[IBIS Ver]   4.2
[File Name]  stm32f2_lqfp100.ibs
[File Rev]   1.0
[Date]   31-Aug-2011
[Source]   STMicroelectronics NV
[Notes]   The I/O models have been made by simulation and qualified
   with recomandation of QualityIBIS flow.
   Some Models, library and pin names may be modified.
   Details of modified names can be found below.
ORIGINAL NAME   ::  MODIFIED NAME   :: COMMENTS(if any)
IO8USB_LSFS_OTG_FT  ::  IO8USB_LSFS_OTG_FT_USB   :: Model in USB mode.
IO8USB_LSFS_OTG_FT  ::  IO8USB_LSFS_OTG_FT_NON_USB_DNV33  :: Model in other than USB mode & pad pin = DNV33
IO8USB_LSFS_OTG_FT  ::  IO8USB_LSFS_OTG_FT_NON_USB_DPV33  :: Model in other than USB mode & pad pin = DPV33
[Disclaimer] These IBIS models are the proprietary information of
   STMicroelectronics and are disclosed to users solely for
   modeling and simulation purposes. No further license is
   implied. All warranties express, implied, or statutory,
   including any implied warranty of fitness for a particular
   purpose or implied warranty against infringement, are
   hereby disclaimed. STMicroelectronics reserves the right
   to change the IBIS models at any time and without notice.
[Copyright]  (c) STMicroelectronics
   All rights reserved. Reproduction in whole or part is prohibited
   without the written consent of the copyright holder.
[Component]  STM32F2_LQFP100
[Manufacturer] STMicroelectronics NV
[Package]
| variable   typ   min   max
R_pkg   0.000mOhm   0.000mOhm   0.000mOhm
L_pkg   0.000nH   0.000nH   0.000nH
C_pkg   0.000pF   0.000pF   0.000pF
[Pin]   signal_name   model_name
1 PE2 IO8PROG2M25M50M100M_ARSUDQ_FT
2 PE3 IO8PROG2M25M50M100M_ARSUDQ_FT
3 PE4 IO8PROG2M25M50M100M_ARSUDQ_FT
4 PE5 IO8PROG2M25M50M100M_ARSUDQ_FT
5 PE6 IO8PROG2M25M50M100M_ARSUDQ_FT
|6 VBAT VDD33IOSWCO_MOSSWI_FT
7 PC13 IO8PROG2M25M50M100M_ARWSUDQ_FT_V33
8 PC14 IO8PROG2M25M50M100M_ARWSUDQ_FT
9 PC15 IO8PROG2M25M50M100M_ARSUDQ_FT
|10 VSS_5 VSSIOCO
|11 VDD_5 VDD33IOCO
12 PH0 IO8PROG2M25M50M100M_ARSUDQ_FT
13 PH1 IO8PROG2M25M50M100M_ARSUDQ_FT
|14 NRST RESET
15 PC0 IO8PROG2M25M50M100M_AR3WSUDQ_FT
16 PC1 IO8PROG2M25M50M100M_AR3WSUDQ_FT
17 PC2 IO8PROG2M25M50M100M_AR3WSUDQ_FT
18 PC3 IO8PROG2M25M50M100M_AR3WSUDQ_FT
|19 VDD_12 VDD33IOCO_VSSIOCO_MOSSWI_FT
|20 VSSA VSSCO
|21 VREF+ VDD33CO
|22 VDDA VDD33CO
23 PA0 IO8PROG2M25M50M100M_AR3WSUDQ_FT_V33
24 PA1 IO8PROG2M25M50M100M_AR3WSUDQ_FT
25 PA2 IO8PROG2M25M50M100M_AR3WSUDQ_FT
26 PA3 IO8PROG2M25M50M100M_AR3WSUDQ_FT
|27 VSS_4 VSSIOCO
|28 VDD_4 VDD33IOCO
29 PA4 IO8PROG2M25M50M100M_AR3WSUDQ_FT
30 PA5 IO8PROG2M25M50M100M_AR3WSUDQ_FT
31 PA6 IO8PROG2M25M50M100M_AR3WSUDQ_FT
32 PA7 IO8PROG2M25M50M100M_AR3WSUDQ_FT
33 PC4 IO8PROG2M25M50M100M_AR3WSUDQ_FT
34 PC5 IO8PROG2M25M50M100M_AR3WSUDQ_FT
35 PB0 IO8PROG2M25M50M100M_AR3WSUDQ_FT
36 PB1 IO8PROG2M25M50M100M_AR3WSUDQ_FT
37 PB2 IO8PROG2M25M50M100M_AR3WSUDQ_FT
38 PE7 IO8PROG2M25M50M100M_ARSUDQ_FT
39 PE8 IO8PROG2M25M50M100M_ARSUDQ_FT
40 PE9 IO8PROG2M25M50M100M_ARSUDQ_FT
41 PE10 IO8PROG2M25M50M100M_ARSUDQ_FT
42 PE11 IO8PROG2M25M50M100M_ARSUDQ_FT
43 PE12 IO8PROG2M25M50M100M_ARSUDQ_FT
44 PE13 IO8PROG2M25M50M100M_ARSUDQ_FT
45 PE14 IO8PROG2M25M50M100M_ARSUDQ_FT
46 PE15 IO8PROG2M25M50M100M_ARSUDQ_FT
47 PB10 IO8PROG2M25M50M100M_ARSUDQ_I2CIN_FT
48 PB11 IO8PROG2M25M50M100M_ARSUDQ_I2CIN_FT
|49 VCAP1_0
|50 VDD_1
51 PB12 IO8USB_ID_OTG_FT
52 PB13 IO8USB_VBUS_OTG_FT
|53 PA11 IO8USB_LSFS_OTG_FT_USB
53 PA11 IO8USB_LSFS_OTG_FT_NON_USB_DNV33
|54 PA12 IO8USB_LSFS_OTG_FT_USB
54 PA12 IO8USB_LSFS_OTG_FT_NON_USB_DPV33
55 PD8 IO8PROG2M25M50M100M_ARSUDQ_FT
56 PD9 IO8PROG2M25M50M100M_ARSUDQ_FT
57 PD10 IO8PROG2M25M50M100M_ARSUDQ_FT
58 PD11 IO8PROG2M25M50M100M_ARSUDQ_FT
59 PD12 IO8PROG2M25M50M100M_ARSUDQ_FT
60 PD13 IO8PROG2M25M50M100M_ARSUDQ_FT
61 PD14 IO8PROG2M25M50M100M_ARSUDQ_FT
62 PD15 IO8PROG2M25M50M100M_ARSUDQ_FT
63 PC6 IO8PROG2M25M50M100M_ARSUDQ_FT
64 PC7 IO8PROG2M25M50M100M_ARSUDQ_FT
65 PC8 IO8PROG2M25M50M100M_ARSUDQ_FT
66 PC9 IO8PROG2M25M50M100M_ARSUDQ_I2CIN_FT
67 PA8 IO8PROG2M25M50M100M_ARSUDQ_I2CIN_FT
68 PA9 IO8USB_VBUS_OTG_FT
69 PA10 IO8USB_ID_OTG_FT
70 PA11 IO8USB_LSFS_OTG_FT_USB
|70 PA11 IO8USB_LSFS_OTG_FT_NON_USB_DNV33
71 PA12 IO8USB_LSFS_OTG_FT_USB
|71 PA12 IO8USB_LSFS_OTG_FT_NON_USB_DPV33
72 PA13 IO8PROG2M25M50M100M_ARSUDQ_FT
|73 VCAP2
|74 VSS_2
|75 VDD_2
76 PA14 IO8PROG2M25M50M100M_ARSUDQ_FT
77 PA15 IO8PROG2M25M50M100M_AR3WSUDQ_FT
78 PC10 IO8PROG2M25M50M100M_ARSUDQ_FT
79 PC11 IO8PROG2M25M50M100M_ARSUDQ_FT
80 PC12 IO8PROG2M25M50M100M_ARSUDQ_FT
81 PD0 IO8PROG2M25M50M100M_ARSUDQ_FT
82 PD1 IO8PROG2M25M50M100M_ARSUDQ_FT
83 PD2 IO8PROG2M25M50M100M_ARSUDQ_FT
84 PD3 IO8PROG2M25M50M100M_ARSUDQ_FT
85 PD4 IO8PROG2M25M50M100M_ARSUDQ_FT
86 PD5 IO8PROG2M25M50M100M_ARSUDQ_FT
87 PD6 IO8PROG2M25M50M100M_ARSUDQ_FT
88 PD7 IO8PROG2M25M50M100M_ARSUDQ_FT
89 PB3 IO8PROG2M25M50M100M_ARSUDQ_FT
90 PB4 IO8PROG2M25M50M100M_ARSUDQ_FT
91 PB5 IO8PROG2M25M50M100M_AR3WSUDQ_FT
92 PB6 IO8PROG2M25M50M100M_ARSUDQ_I2CIN_FT
93 PB7 IO8PROG2M25M50M100M_ARSUDQ_I2CIN_FT
94 BOOT0 VPP_TEST_HV
95 PB8 IO8PROG2M25M50M100M_ARSUDQ_I2CIN_FT
96 PB9 IO8PROG2M25M50M100M_ARSUDQ_I2CIN_FT
97 PE0 IO8PROG2M25M50M100M_ARSUDQ_FT
98 PE1 IO8PROG2M25M50M100M_ARSUDQ_FT
|99 NC
|100 VDD_3  VDD33CO
[Diff Pin]  inv_pin   vdiff tdelay_typ tdelay_min tdelay_max
|53 54 200mV 0  0 0
70 71 200mV 0  0 0
[Model Selector] IO8PROG2M25M50M100M_AR3WSUDQ_FT_V33
IO8PROG2M25M50M100M_AR3WSUDQ_DRV_V33_00   DRIVER MODEL  : SPEEDAV33=0 SPEEDBV33=0
IO8PROG2M25M50M100M_AR3WSUDQ_DRV_V33_01   DRIVER MODEL  : SPEEDAV33=0 SPEEDBV33=1
IO8PROG2M25M50M100M_AR3WSUDQ_DRV_V33_10   DRIVER MODEL  : SPEEDAV33=1 SPEEDBV33=0
IO8PROG2M25M50M100M_AR3WSUDQ_DRV_V33_11   DRIVER MODEL  : SPEEDAV33=1 SPEEDBV33=1
IO8PROG2M25M50M100M_AR3WSUDQ_RCV_V33_0   CMOS RECIEVER : ENHYSV33=0  OUTPUT=ZIV33
IO8PROG2M25M50M100M_AR3WSUDQ_RCV_V33_0_T  TTL  RECIEVER : ENHYSV33=0  OUTPUT=ZIV33
IO8PROG2M25M50M100M_AR3WSUDQ_RCV_V33_1   CMOS RECIEVER : ENHYSV33=1  OUTPUT=ZIV33
IO8PROG2M25M50M100M_AR3WSUDQ_RCV_V33_1_T  TTL  RECIEVER : ENHYSV33=1  OUTPUT=ZIV33
[Model Selector] IO8PROG2M25M50M100M_AR3WSUDQ_FT
IO8PROG2M25M50M100M_AR3WSUDQ_FT_DRV_00   DRIVER MODEL  : SPEEDAV12=0 SPEEDBV12=0
IO8PROG2M25M50M100M_AR3WSUDQ_FT_DRV_01   DRIVER MODEL  : SPEEDAV12=0 SPEEDBV12=1
IO8PROG2M25M50M100M_AR3WSUDQ_FT_DRV_10   DRIVER MODEL  : SPEEDAV12=1 SPEEDBV12=0
IO8PROG2M25M50M100M_AR3WSUDQ_FT_DRV_11   DRIVER MODEL  : SPEEDAV12=1 SPEEDBV12=1
IO8PROG2M25M50M100M_AR3WSUDQ_FT_RCV_00   CMOS RECIEVER : ENHYSV12=0  OUTPUT=ZIV12
IO8PROG2M25M50M100M_AR3WSUDQ_FT_RCV_00_T  TTL  RECIEVER : ENHYSV12=0  OUTPUT=ZIV12
IO8PROG2M25M50M100M_AR3WSUDQ_FT_RCV_01   CMOS RECIEVER : ENHYSV12=0  OUTPUT=ZIV33
IO8PROG2M25M50M100M_AR3WSUDQ_FT_RCV_01_T  TTL  RECIEVER : ENHYSV12=0  OUTPUT=ZIV33
IO8PROG2M25M50M100M_AR3WSUDQ_FT_RCV_10   CMOS RECIEVER : ENHYSV12=1  OUTPUT=ZIV12
IO8PROG2M25M50M100M_AR3WSUDQ_FT_RCV_10_T  TTL  RECIEVER : ENHYSV12=1  OUTPUT=ZIV12
IO8PROG2M25M50M100M_AR3WSUDQ_FT_RCV_11   CMOS RECIEVER : ENHYSV12=1  OUTPUT=ZIV33
IO8PROG2M25M50M100M_AR3WSUDQ_FT_RCV_11_T  TTL  RECIEVER : ENHYSV12=1  OUTPUT=ZIV33
[Model Selector] IO8PROG2M25M50M100M_ARSUDQ_FT
IO8PROG2M25M50M100M_ARSUDQ_FT_DRV_00   DRIVER MODEL  : SPEEDAV12=0 SPEEDBV12=0
IO8PROG2M25M50M100M_ARSUDQ_FT_DRV_01   DRIVER MODEL  : SPEEDAV12=0 SPEEDBV12=1
IO8PROG2M25M50M100M_ARSUDQ_FT_DRV_10   DRIVER MODEL  : SPEEDAV12=1 SPEEDBV12=0
IO8PROG2M25M50M100M_ARSUDQ_FT_DRV_11   DRIVER MODEL  : SPEEDAV12=1 SPEEDBV12=1
IO8PROG2M25M50M100M_ARSUDQ_FT_RCV_00   CMOS RECIEVER : ENHYSV12=0  OUTPUT=ZIV12
IO8PROG2M25M50M100M_ARSUDQ_FT_RCV_00_T   TTL  RECIEVER : ENHYSV12=0  OUTPUT=ZIV12
IO8PROG2M25M50M100M_ARSUDQ_FT_RCV_01   CMOS RECIEVER : ENHYSV12=0  OUTPUT=ZIV33
IO8PROG2M25M50M100M_ARSUDQ_FT_RCV_01_T   TTL  RECIEVER : ENHYSV12=0  OUTPUT=ZIV33
IO8PROG2M25M50M100M_ARSUDQ_FT_RCV_10   CMOS RECIEVER : ENHYSV12=1  OUTPUT=ZIV12
IO8PROG2M25M50M100M_ARSUDQ_FT_RCV_10_T   TTL  RECIEVER : ENHYSV12=1  OUTPUT=ZIV12
IO8PROG2M25M50M100M_ARSUDQ_FT_RCV_11   CMOS RECIEVER : ENHYSV12=1  OUTPUT=ZIV33
IO8PROG2M25M50M100M_ARSUDQ_FT_RCV_11_T   TTL  RECIEVER : ENHYSV12=1  OUTPUT=ZIV33
[Model Selector] IO8PROG2M25M50M100M_ARSUDQ_I2CIN_FT
IO8PROG2M25M50M100M_ARSUDQ_I2CIN_DRV_00   DRIVER MODEL  : SPEEDAV12=0 SPEEDBV12=0
IO8PROG2M25M50M100M_ARSUDQ_I2CIN_DRV_01   DRIVER MODEL  : SPEEDAV12=0 SPEEDBV12=1
IO8PROG2M25M50M100M_ARSUDQ_I2CIN_DRV_10   DRIVER MODEL  : SPEEDAV12=1 SPEEDBV12=0
IO8PROG2M25M50M100M_ARSUDQ_I2CIN_DRV_11   DRIVER MODEL  : SPEEDAV12=1 SPEEDBV12=1
IO8PROG2M25M50M100M_I2CIN_RCV_ZII2C_00   CMOS RECIEVER : TESTI2CV12=0  HSFSV12=0
IO8PROG2M25M50M100M_I2CIN_RCV_ZII2C_00_T   TTL  RECIEVER : TESTI2CV12=0  HSFSV12=0
IO8PROG2M25M50M100M_I2CIN_RCV_ZII2C_01   CMOS RECIEVER : TESTI2CV12=0  HSFSV12=1
IO8PROG2M25M50M100M_I2CIN_RCV_ZII2C_01_T   TTL  RECIEVER : TESTI2CV12=0  HSFSV12=1
IO8PROG2M25M50M100M_I2CIN_RCV_ZII2C_10   CMOS RECIEVER : TESTI2CV12=1  HSFSV12=0
IO8PROG2M25M50M100M_I2CIN_RCV_ZII2C_10_T   TTL  RECIEVER : TESTI2CV12=1  HSFSV12=0
IO8PROG2M25M50M100M_I2CIN_RCV_ZII2C_11   CMOS RECIEVER : TESTI2CV12=1  HSFSV12=1
IO8PROG2M25M50M100M_I2CIN_RCV_ZII2C_11_T   TTL  RECIEVER : TESTI2CV12=1  HSFSV12=1
IO8PROG2M25M50M100M_I2CIN_RCV_ZIV12_0   CMOS RECIEVER : ENHYSV12=0  OUTPUT=ZIV12
IO8PROG2M25M50M100M_I2CIN_RCV_ZIV12_0_T   TTL  RECIEVER : ENHYSV12=0  OUTPUT=ZIV12
IO8PROG2M25M50M100M_I2CIN_RCV_ZIV12_1   CMOS RECIEVER : ENHYSV12=1  OUTPUT=ZIV12
IO8PROG2M25M50M100M_I2CIN_RCV_ZIV12_1_T   TTL  RECIEVER : ENHYSV12=1  OUTPUT=ZIV12
IO8PROG2M25M50M100M_I2CIN_RCV_ZIV33_0   CMOS RECIEVER : ENHYSV12=0  OUTPUT=ZIV33
IO8PROG2M25M50M100M_I2CIN_RCV_ZIV33_0_T   TTL  RECIEVER : ENHYSV12=0  OUTPUT=ZIV33
IO8PROG2M25M50M100M_I2CIN_RCV_ZIV33_1   CMOS RECIEVER : ENHYSV12=1  OUTPUT=ZIV33
IO8PROG2M25M50M100M_I2CIN_RCV_ZIV33_1_T   TTL  RECIEVER : ENHYSV12=1  OUTPUT=ZIV33
[Model Selector] IO8PROG2M25M50M100M_ARWSUDQ_FT_V33
IO8PROG2M25M50M100M_ARWSUDQ_DRV_V33_00   DRIVER MODEL  : SPEEDAV33=0 SPEEDBV33=0
IO8PROG2M25M50M100M_ARWSUDQ_DRV_V33_01   DRIVER MODEL  : SPEEDAV33=0 SPEEDBV33=1
IO8PROG2M25M50M100M_ARWSUDQ_DRV_V33_10   DRIVER MODEL  : SPEEDAV33=1 SPEEDBV33=0
IO8PROG2M25M50M100M_ARWSUDQ_DRV_V33_11   DRIVER MODEL  : SPEEDAV33=1 SPEEDBV33=1
IO8PROG2M25M50M100M_ARWSUDQ_RCV_V33_0   CMOS RECIEVER : ENHYSV33=0  OUTPUT=ZIV33
IO8PROG2M25M50M100M_ARWSUDQ_RCV_V33_0_T   TTL  RECIEVER : ENHYSV33=0  OUTPUT=ZIV33
IO8PROG2M25M50M100M_ARWSUDQ_RCV_V33_1   CMOS RECIEVER : ENHYSV33=1  OUTPUT=ZIV33
IO8PROG2M25M50M100M_ARWSUDQ_RCV_V33_1_T   TTL  RECIEVER : ENHYSV33=1  OUTPUT=ZIV33
[Model Selector] IO8PROG2M25M50M100M_ARWSUDQ_FT
IO8PROG2M25M50M100M_ARWSUDQ_FT_DRV_00   DRIVER MODEL  : SPEEDAV12=0 SPEEDBV12=0
IO8PROG2M25M50M100M_ARWSUDQ_FT_DRV_01   DRIVER MODEL  : SPEEDAV12=0 SPEEDBV12=1
IO8PROG2M25M50M100M_ARWSUDQ_FT_DRV_10   DRIVER MODEL  : SPEEDAV12=1 SPEEDBV12=0
IO8PROG2M25M50M100M_ARWSUDQ_FT_DRV_11   DRIVER MODEL  : SPEEDAV12=1 SPEEDBV12=1
IO8PROG2M25M50M100M_ARWSUDQ_FT_RCV_00   CMOS RECIEVER : ENHYSV12=0  OUTPUT=ZIV12
IO8PROG2M25M50M100M_ARWSUDQ_FT_RCV_00_T   TTL  RECIEVER : ENHYSV12=0  OUTPUT=ZIV12
IO8PROG2M25M50M100M_ARWSUDQ_FT_RCV_01   CMOS RECIEVER : ENHYSV12=0  OUTPUT=ZIV33
IO8PROG2M25M50M100M_ARWSUDQ_FT_RCV_01_T   TTL  RECIEVER : ENHYSV12=0  OUTPUT=ZIV33
IO8PROG2M25M50M100M_ARWSUDQ_FT_RCV_10   CMOS RECIEVER : ENHYSV12=1  OUTPUT=ZIV12
IO8PROG2M25M50M100M_ARWSUDQ_FT_RCV_10_T   TTL  RECIEVER : ENHYSV12=1  OUTPUT=ZIV12
IO8PROG2M25M50M100M_ARWSUDQ_FT_RCV_11   CMOS RECIEVER : ENHYSV12=1  OUTPUT=ZIV33
IO8PROG2M25M50M100M_ARWSUDQ_FT_RCV_11_T   TTL  RECIEVER : ENHYSV12=1  OUTPUT=ZIV33
[Model Selector] IO8USB_ID_OTG_FT
IO8USB_ID_OTG_FT_DRV_00   DRIVER MODEL  : SPEEDAV12=0 SPEEDBV12=0
IO8USB_ID_OTG_FT_DRV_01   DRIVER MODEL  : SPEEDAV12=0 SPEEDBV12=1
IO8USB_ID_OTG_FT_DRV_10   DRIVER MODEL  : SPEEDAV12=1 SPEEDBV12=0
IO8USB_ID_OTG_FT_DRV_11   DRIVER MODEL  : SPEEDAV12=1 SPEEDBV12=1
IO8USB_ID_OTG_FT_RCV_00   CMOS RECIEVER : ENHYSV12=0  OUTPUT=ZIV12
IO8USB_ID_OTG_FT_RCV_00_T   TTL  RECIEVER : ENHYSV12=0  OUTPUT=ZIV12
IO8USB_ID_OTG_FT_RCV_01   CMOS RECIEVER : ENHYSV12=0  OUTPUT=ZIV33
IO8USB_ID_OTG_FT_RCV_01_T   TTL  RECIEVER : ENHYSV12=0  OUTPUT=ZIV33
IO8USB_ID_OTG_FT_RCV_10   CMOS RECIEVER : ENHYSV12=1  OUTPUT=ZIV12
IO8USB_ID_OTG_FT_RCV_10_T   TTL  RECIEVER : ENHYSV12=1  OUTPUT=ZIV12
IO8USB_ID_OTG_FT_RCV_11   CMOS RECIEVER : ENHYSV12=1  OUTPUT=ZIV33
IO8USB_ID_OTG_FT_RCV_11_T   TTL  RECIEVER : ENHYSV12=1  OUTPUT=ZIV33
[Model Selector] IO8USB_LSFS_OTG_FT_USB
IO8USB_LSFS_OTG_FT_DRV_USB_0   DRIVER : USBLSFSV12=0 ENUSBV12=0
IO8USB_LSFS_OTG_FT_DRV_USB_1   DRIVER : USBLSFSV12=1 ENUSBV12=0
IO8USB_LSFS_OTG_FT_RCV_USB   USB  RECIEVER : ENHYSV12=1  OUTPUT=USBZIV12
[Model Selector] IO8USB_LSFS_OTG_FT_NON_USB_DNV33
IO8USB_LSFS_OTG_FT_DRV_IO8_DNV33_00   DRIVER : SPEEDAV12=0 SPEEDBV12=0 ENUSBV12=1
IO8USB_LSFS_OTG_FT_DRV_IO8_DNV33_01   DRIVER : SPEEDAV12=0 SPEEDBV12=1 ENUSBV12=1
IO8USB_LSFS_OTG_FT_DRV_IO8_DNV33_10   DRIVER : SPEEDAV12=1 SPEEDBV12=0 ENUSBV12=1
IO8USB_LSFS_OTG_FT_DRV_IO8_DNV33_11   DRIVER : SPEEDAV12=1 SPEEDBV12=1 ENUSBV12=1
IO8USB_LSFS_OTG_FT_RCV_IO8_ZINV12_0   CMOS RECIEVER : ENHYSV12=0  OUTPUT=ZIV12
IO8USB_LSFS_OTG_FT_RCV_IO8_ZINV12_0_T  TTL  RECIEVER : ENHYSV12=0  OUTPUT=ZIV12
IO8USB_LSFS_OTG_FT_RCV_IO8_ZINV12_1   CMOS RECIEVER : ENHYSV12=1  OUTPUT=ZIV12
IO8USB_LSFS_OTG_FT_RCV_IO8_ZINV12_1_T  TTL  RECIEVER : ENHYSV12=1  OUTPUT=ZIV12
IO8USB_LSFS_OTG_FT_RCV_IO8_ZINV33_0   CMOS RECIEVER : ENHYSV12=0  OUTPUT=ZIV33
IO8USB_LSFS_OTG_FT_RCV_IO8_ZINV33_0_T  TTL  RECIEVER : ENHYSV12=0  OUTPUT=ZIV33
IO8USB_LSFS_OTG_FT_RCV_IO8_ZINV33_1   CMOS RECIEVER : ENHYSV12=1  OUTPUT=ZIV33
IO8USB_LSFS_OTG_FT_RCV_IO8_ZINV33_1_T  TTL  RECIEVER : ENHYSV12=1  OUTPUT=ZIV33
[Model Selector] IO8USB_LSFS_OTG_FT_NON_USB_DPV33
IO8USB_LSFS_OTG_FT_DRV_IO8_DPV33_00   DRIVER : SPEEDAV12=0 SPEEDBV12=0 ENUSBV12=1
IO8USB_LSFS_OTG_FT_DRV_IO8_DPV33_01   DRIVER : SPEEDAV12=0 SPEEDBV12=1 ENUSBV12=1
IO8USB_LSFS_OTG_FT_DRV_IO8_DPV33_10   DRIVER : SPEEDAV12=1 SPEEDBV12=0 ENUSBV12=1
IO8USB_LSFS_OTG_FT_DRV_IO8_DPV33_11   DRIVER : SPEEDAV12=1 SPEEDBV12=1 ENUSBV12=1
IO8USB_LSFS_OTG_FT_RCV_IO8_ZIPV12_0   CMOS RECIEVER : ENHYSV12=0  OUTPUT=ZIV12
IO8USB_LSFS_OTG_FT_RCV_IO8_ZIPV12_0_T  TTL  RECIEVER : ENHYSV12=0  OUTPUT=ZIV12
IO8USB_LSFS_OTG_FT_RCV_IO8_ZIPV12_1   CMOS RECIEVER : ENHYSV12=1  OUTPUT=ZIV12
IO8USB_LSFS_OTG_FT_RCV_IO8_ZIPV12_1_T  TTL  RECIEVER : ENHYSV12=1  OUTPUT=ZIV12
IO8USB_LSFS_OTG_FT_RCV_IO8_ZIPV33_0   CMOS RECIEVER : ENHYSV12=0  OUTPUT=ZIV33
IO8USB_LSFS_OTG_FT_RCV_IO8_ZIPV33_0_T  TTL  RECIEVER : ENHYSV12=0  OUTPUT=ZIV33
IO8USB_LSFS_OTG_FT_RCV_IO8_ZIPV33_1   CMOS RECIEVER : ENHYSV12=1  OUTPUT=ZIV33
IO8USB_LSFS_OTG_FT_RCV_IO8_ZIPV33_1_T  TTL  RECIEVER : ENHYSV12=1  OUTPUT=ZIV33
[Model Selector] IO8USB_VBUS_OTG_FT
IO8USB_VBUS_OTG_FT_DRV_00   DRIVER MODEL  : SPEEDAV12=0 SPEEDBV12=0
IO8USB_VBUS_OTG_FT_DRV_01   DRIVER MODEL  : SPEEDAV12=0 SPEEDBV12=1
IO8USB_VBUS_OTG_FT_DRV_10   DRIVER MODEL  : SPEEDAV12=1 SPEEDBV12=0
IO8USB_VBUS_OTG_FT_DRV_11   DRIVER MODEL  : SPEEDAV12=1 SPEEDBV12=1
IO8USB_VBUS_OTG_FT_RCV_00   CMOS RECIEVER : ENHYSV12=0  OUTPUT=ZIV12
IO8USB_VBUS_OTG_FT_RCV_00_T   TTL  RECIEVER : ENHYSV12=0  OUTPUT=ZIV12
IO8USB_VBUS_OTG_FT_RCV_01   CMOS RECIEVER : ENHYSV12=0  OUTPUT=ZIV33
IO8USB_VBUS_OTG_FT_RCV_01_T   TTL  RECIEVER : ENHYSV12=0  OUTPUT=ZIV33
IO8USB_VBUS_OTG_FT_RCV_10   CMOS RECIEVER : ENHYSV12=1  OUTPUT=ZIV12
IO8USB_VBUS_OTG_FT_RCV_10_T   TTL  RECIEVER : ENHYSV12=1  OUTPUT=ZIV12
IO8USB_VBUS_OTG_FT_RCV_11   CMOS RECIEVER : ENHYSV12=1  OUTPUT=ZIV33
IO8USB_VBUS_OTG_FT_RCV_11_T   TTL  RECIEVER : ENHYSV12=1  OUTPUT=ZIV33
[Model Selector] VPP_TEST_HV
VPP_TEST_HV_00   CMOS RECIEVER : ENHYSV12=0  OUTPUT=ZIV12
VPP_TEST_HV_00_T   TTL  RECIEVER : ENHYSV12=0  OUTPUT=ZIV12
VPP_TEST_HV_01   CMOS RECIEVER : ENHYSV12=0  OUTPUT=ZIV33
VPP_TEST_HV_01_T   TTL  RECIEVER : ENHYSV12=0  OUTPUT=ZIV33
VPP_TEST_HV_10   CMOS RECIEVER : ENHYSV12=1  OUTPUT=ZIV12
VPP_TEST_HV_10_T   TTL  RECIEVER : ENHYSV12=1  OUTPUT=ZIV12
VPP_TEST_HV_11   CMOS RECIEVER : ENHYSV12=1  OUTPUT=ZIV33
VPP_TEST_HV_11_T   TTL  RECIEVER : ENHYSV12=1  OUTPUT=ZIV33
| Models and submodels in the file (131): IO8PROG2M25M50M100M_AR3WSUDQ_DRV_V33_00 (3-state), IO8PROG2M25M50M100M_AR3WSUDQ_DRV_V33_01 (3-state), IO8PROG2M25M50M100M_AR3WSUDQ_DRV_V33_10 (3-state), IO8PROG2M25M50M100M_AR3WSUDQ_DRV_V33_11 (3-state), IO8PROG2M25M50M100M_AR3WSUDQ_FT_DRV_00 (3-state), IO8PROG2M25M50M100M_AR3WSUDQ_FT_DRV_01 (3-state), IO8PROG2M25M50M100M_AR3WSUDQ_FT_DRV_10 (3-state), IO8PROG2M25M50M100M_AR3WSUDQ_FT_DRV_11 (3-state), IO8PROG2M25M50M100M_AR3WSUDQ_FT_RCV_00 (Input), IO8PROG2M25M50M100M_AR3WSUDQ_FT_RCV_00_T (Input), IO8PROG2M25M50M100M_AR3WSUDQ_FT_RCV_01 (Input), IO8PROG2M25M50M100M_AR3WSUDQ_FT_RCV_01_T (Input), IO8PROG2M25M50M100M_AR3WSUDQ_FT_RCV_10 (Input), IO8PROG2M25M50M100M_AR3WSUDQ_FT_RCV_10_T (Input), IO8PROG2M25M50M100M_AR3WSUDQ_FT_RCV_11 (Input), IO8PROG2M25M50M100M_AR3WSUDQ_FT_RCV_11_T (Input), IO8PROG2M25M50M100M_AR3WSUDQ_RCV_V33_0 (Input), IO8PROG2M25M50M100M_AR3WSUDQ_RCV_V33_0_T (Input), IO8PROG2M25M50M100M_AR3WSUDQ_RCV_V33_1 (Input), IO8PROG2M25M50M100M_AR3WSUDQ_RCV_V33_1_T (Input), IO8PROG2M25M50M100M_ARSUDQ_FT_DRV_00 (3-state), IO8PROG2M25M50M100M_ARSUDQ_FT_DRV_01 (3-state), IO8PROG2M25M50M100M_ARSUDQ_FT_DRV_10 (3-state), IO8PROG2M25M50M100M_ARSUDQ_FT_DRV_11 (3-state), IO8PROG2M25M50M100M_ARSUDQ_FT_RCV_00 (Input), IO8PROG2M25M50M100M_ARSUDQ_FT_RCV_00_T (Input), IO8PROG2M25M50M100M_ARSUDQ_FT_RCV_01 (Input), IO8PROG2M25M50M100M_ARSUDQ_FT_RCV_01_T (Input), IO8PROG2M25M50M100M_ARSUDQ_FT_RCV_10 (Input), IO8PROG2M25M50M100M_ARSUDQ_FT_RCV_10_T (Input), IO8PROG2M25M50M100M_ARSUDQ_FT_RCV_11 (Input), IO8PROG2M25M50M100M_ARSUDQ_FT_RCV_11_T (Input), IO8PROG2M25M50M100M_ARSUDQ_I2CIN_DRV_00 (3-state), IO8PROG2M25M50M100M_ARSUDQ_I2CIN_DRV_01 (3-state), IO8PROG2M25M50M100M_ARSUDQ_I2CIN_DRV_10 (3-state), IO8PROG2M25M50M100M_ARSUDQ_I2CIN_DRV_11 (3-state), IO8PROG2M25M50M100M_ARWSUDQ_DRV_V33_00 (3-state), IO8PROG2M25M50M100M_ARWSUDQ_DRV_V33_01 (3-state), IO8PROG2M25M50M100M_ARWSUDQ_DRV_V33_10 (3-state), IO8PROG2M25M50M100M_ARWSUDQ_DRV_V33_11 (3-state), IO8PROG2M25M50M100M_ARWSUDQ_FT_DRV_00 (3-state), IO8PROG2M25M50M100M_ARWSUDQ_FT_DRV_01 (3-state), IO8PROG2M25M50M100M_ARWSUDQ_FT_DRV_10 (3-state), IO8PROG2M25M50M100M_ARWSUDQ_FT_DRV_11 (3-state), IO8PROG2M25M50M100M_ARWSUDQ_FT_RCV_00 (Input), IO8PROG2M25M50M100M_ARWSUDQ_FT_RCV_00_T (Input), IO8PROG2M25M50M100M_ARWSUDQ_FT_RCV_01 (Input), IO8PROG2M25M50M100M_ARWSUDQ_FT_RCV_01_T (Input), IO8PROG2M25M50M100M_ARWSUDQ_FT_RCV_10 (Input), IO8PROG2M25M50M100M_ARWSUDQ_FT_RCV_10_T (Input), IO8PROG2M25M50M100M_ARWSUDQ_FT_RCV_11 (Input), IO8PROG2M25M50M100M_ARWSUDQ_FT_RCV_11_T (Input), IO8PROG2M25M50M100M_ARWSUDQ_RCV_V33_0 (Input), IO8PROG2M25M50M100M_ARWSUDQ_RCV_V33_0_T (Input), IO8PROG2M25M50M100M_ARWSUDQ_RCV_V33_1 (Input), IO8PROG2M25M50M100M_ARWSUDQ_RCV_V33_1_T (Input), IO8PROG2M25M50M100M_I2CIN_RCV_ZII2C_00 (Input), IO8PROG2M25M50M100M_I2CIN_RCV_ZII2C_00_T (Input), IO8PROG2M25M50M100M_I2CIN_RCV_ZII2C_01 (Input), IO8PROG2M25M50M100M_I2CIN_RCV_ZII2C_01_T (Input), IO8PROG2M25M50M100M_I2CIN_RCV_ZII2C_10 (Input), IO8PROG2M25M50M100M_I2CIN_RCV_ZII2C_10_T (Input), IO8PROG2M25M50M100M_I2CIN_RCV_ZII2C_11 (Input), IO8PROG2M25M50M100M_I2CIN_RCV_ZII2C_11_T (Input), IO8PROG2M25M50M100M_I2CIN_RCV_ZIV12_0 (Input), IO8PROG2M25M50M100M_I2CIN_RCV_ZIV12_0_T (Input), IO8PROG2M25M50M100M_I2CIN_RCV_ZIV12_1 (Input), IO8PROG2M25M50M100M_I2CIN_RCV_ZIV12_1_T (Input), IO8PROG2M25M50M100M_I2CIN_RCV_ZIV33_0 (Input), IO8PROG2M25M50M100M_I2CIN_RCV_ZIV33_0_T (Input), IO8PROG2M25M50M100M_I2CIN_RCV_ZIV33_1 (Input), IO8PROG2M25M50M100M_I2CIN_RCV_ZIV33_1_T (Input), IO8USB_ID_OTG_FT_DRV_00 (3-state), IO8USB_ID_OTG_FT_DRV_01 (3-state), IO8USB_ID_OTG_FT_DRV_10 (3-state), IO8USB_ID_OTG_FT_DRV_11 (3-state), IO8USB_ID_OTG_FT_RCV_00 (Input), IO8USB_ID_OTG_FT_RCV_00_T (Input), IO8USB_ID_OTG_FT_RCV_01 (Input), IO8USB_ID_OTG_FT_RCV_01_T (Input)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
